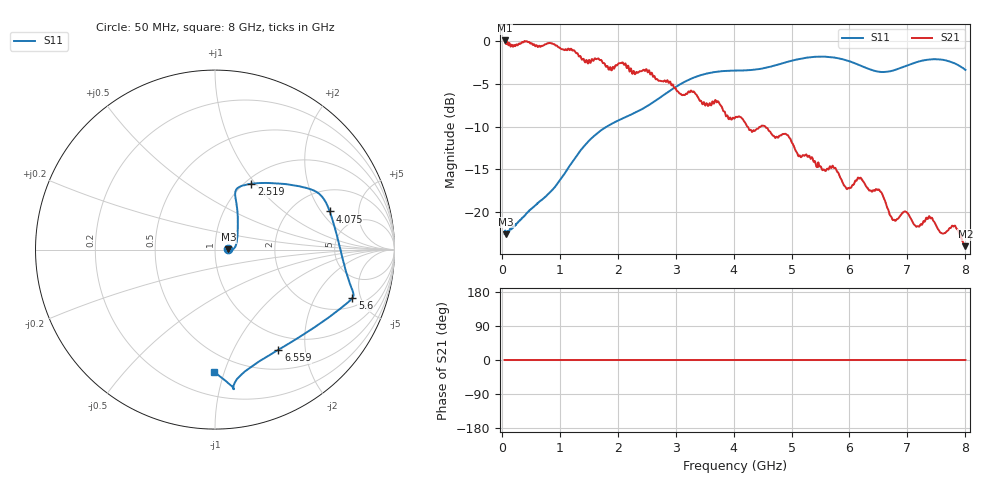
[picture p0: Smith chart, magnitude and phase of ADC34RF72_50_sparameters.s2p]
! Texas Instruments, Inc.
! ADC34RF72 - Single Channel S-Parameters - Fs = 1.5 GSPS, Termination = 50
! Port 1 represents the 50-ohm differential input, Port 2 represents the digital output of the ADC
! freq  magS11  angS11  magS21  angS21  magS12  angS12  magS22  angS22
# Hz S ma R 50
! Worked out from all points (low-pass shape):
!   1601 points, 50 MHz to 8 GHz, reference 50 ohm
!   highest |S21| = 0.10 dB at 54.97 MHz (marker M1); lowest = -24.0 dB at 8 GHz (marker M2)
!   |S21| within 3 dB of the highest: start of sweep to 1.791 GHz; 1.958 GHz to 2.147 GHz (189.2 MHz wide, 9.22 % of centre)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
!   lowest |S11| = -22.6 dB at 74.84 MHz (marker M3), VSWR 1.16, Z = 58 + j0.295 ohm
!   |S11| at or under -10 dB: start of sweep to 1.813 GHz
!   S12 and S22 are empty: the file has one direction only
!   S11 on the Smith chart (normalised r, x): 50 MHz: 1.16, +0.01; 2.519 GHz: 1.07, +0.95; 4.075 GHz: 3.12, +2.43; 5.6 GHz: 2.69, -4.23; 6.559 GHz: 0.77, -1.53; 8 GHz: 0.37, -0.92
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5e7  0.07436 2.0  1 0.0  0 0.0  0 0.0
5.496875e7  0.07572 2.7  1.011 0.0  0 0.0  0 0.0
7.484375e7  0.07427 1.9  0.9643 0.0  0 0.0  0 0.0
8.499688e8  0.1323 22.4  0.9735 0.0  0 0.0  0 0.0
1.376656e9  0.2327 57.3  0.7881 0.0  0 0.0  0 0.0
2.519469e9  0.419 61.1  0.657 0.0  0 0.0  0 0.0
2.703312e9  0.4601 53.8  0.5882 0.0  0 0.0  0 0.0
3.324406e9  0.6142 34.0  0.5034 0.0  0 0.0  0 0.0
4.025e9  0.673 19.9  0.3556 0.0  0 0.0  0 0.0
4.074688e9  0.6738 18.4  0.361 0.0  0 0.0  0 0.0
4.854781e9  0.7447 -10.2  0.2863 0.0  0 0.0  0 0.0
5.351656e9  0.8083 -17.5  0.2091 0.0  0 0.0  0 0.0
5.600094e9  0.8115 -19.3  0.1757 0.0  0 0.0  0 0.0
6.062188e9  0.7501 -28.7  0.1441 0.0  0 0.0  0 0.0
6.559062e9  0.6602 -57.7  0.1286 0.0  0 0.0  0 0.0
6.678312e9  0.6647 -65.6  0.1005 0.0  0 0.0  0 0.0
7.016188e9  0.7261 -79.8  0.09693 0.0  0 0.0  0 0.0
7.170219e9  0.7566 -81.9  0.08231 0.0  0 0.0  0 0.0
7.393812e9  0.7823 -82.4  0.09186 0.0  0 0.0  0 0.0
7.592562e9  0.7805 -82.4  0.075 0.0  0 0.0  0 0.0
7.831062e9  0.7378 -85.0  0.08184 0.0  0 0.0  0 0.0
8e9  0.6797 -90.4  0.06291 0.0  0 0.0  0 0.0
